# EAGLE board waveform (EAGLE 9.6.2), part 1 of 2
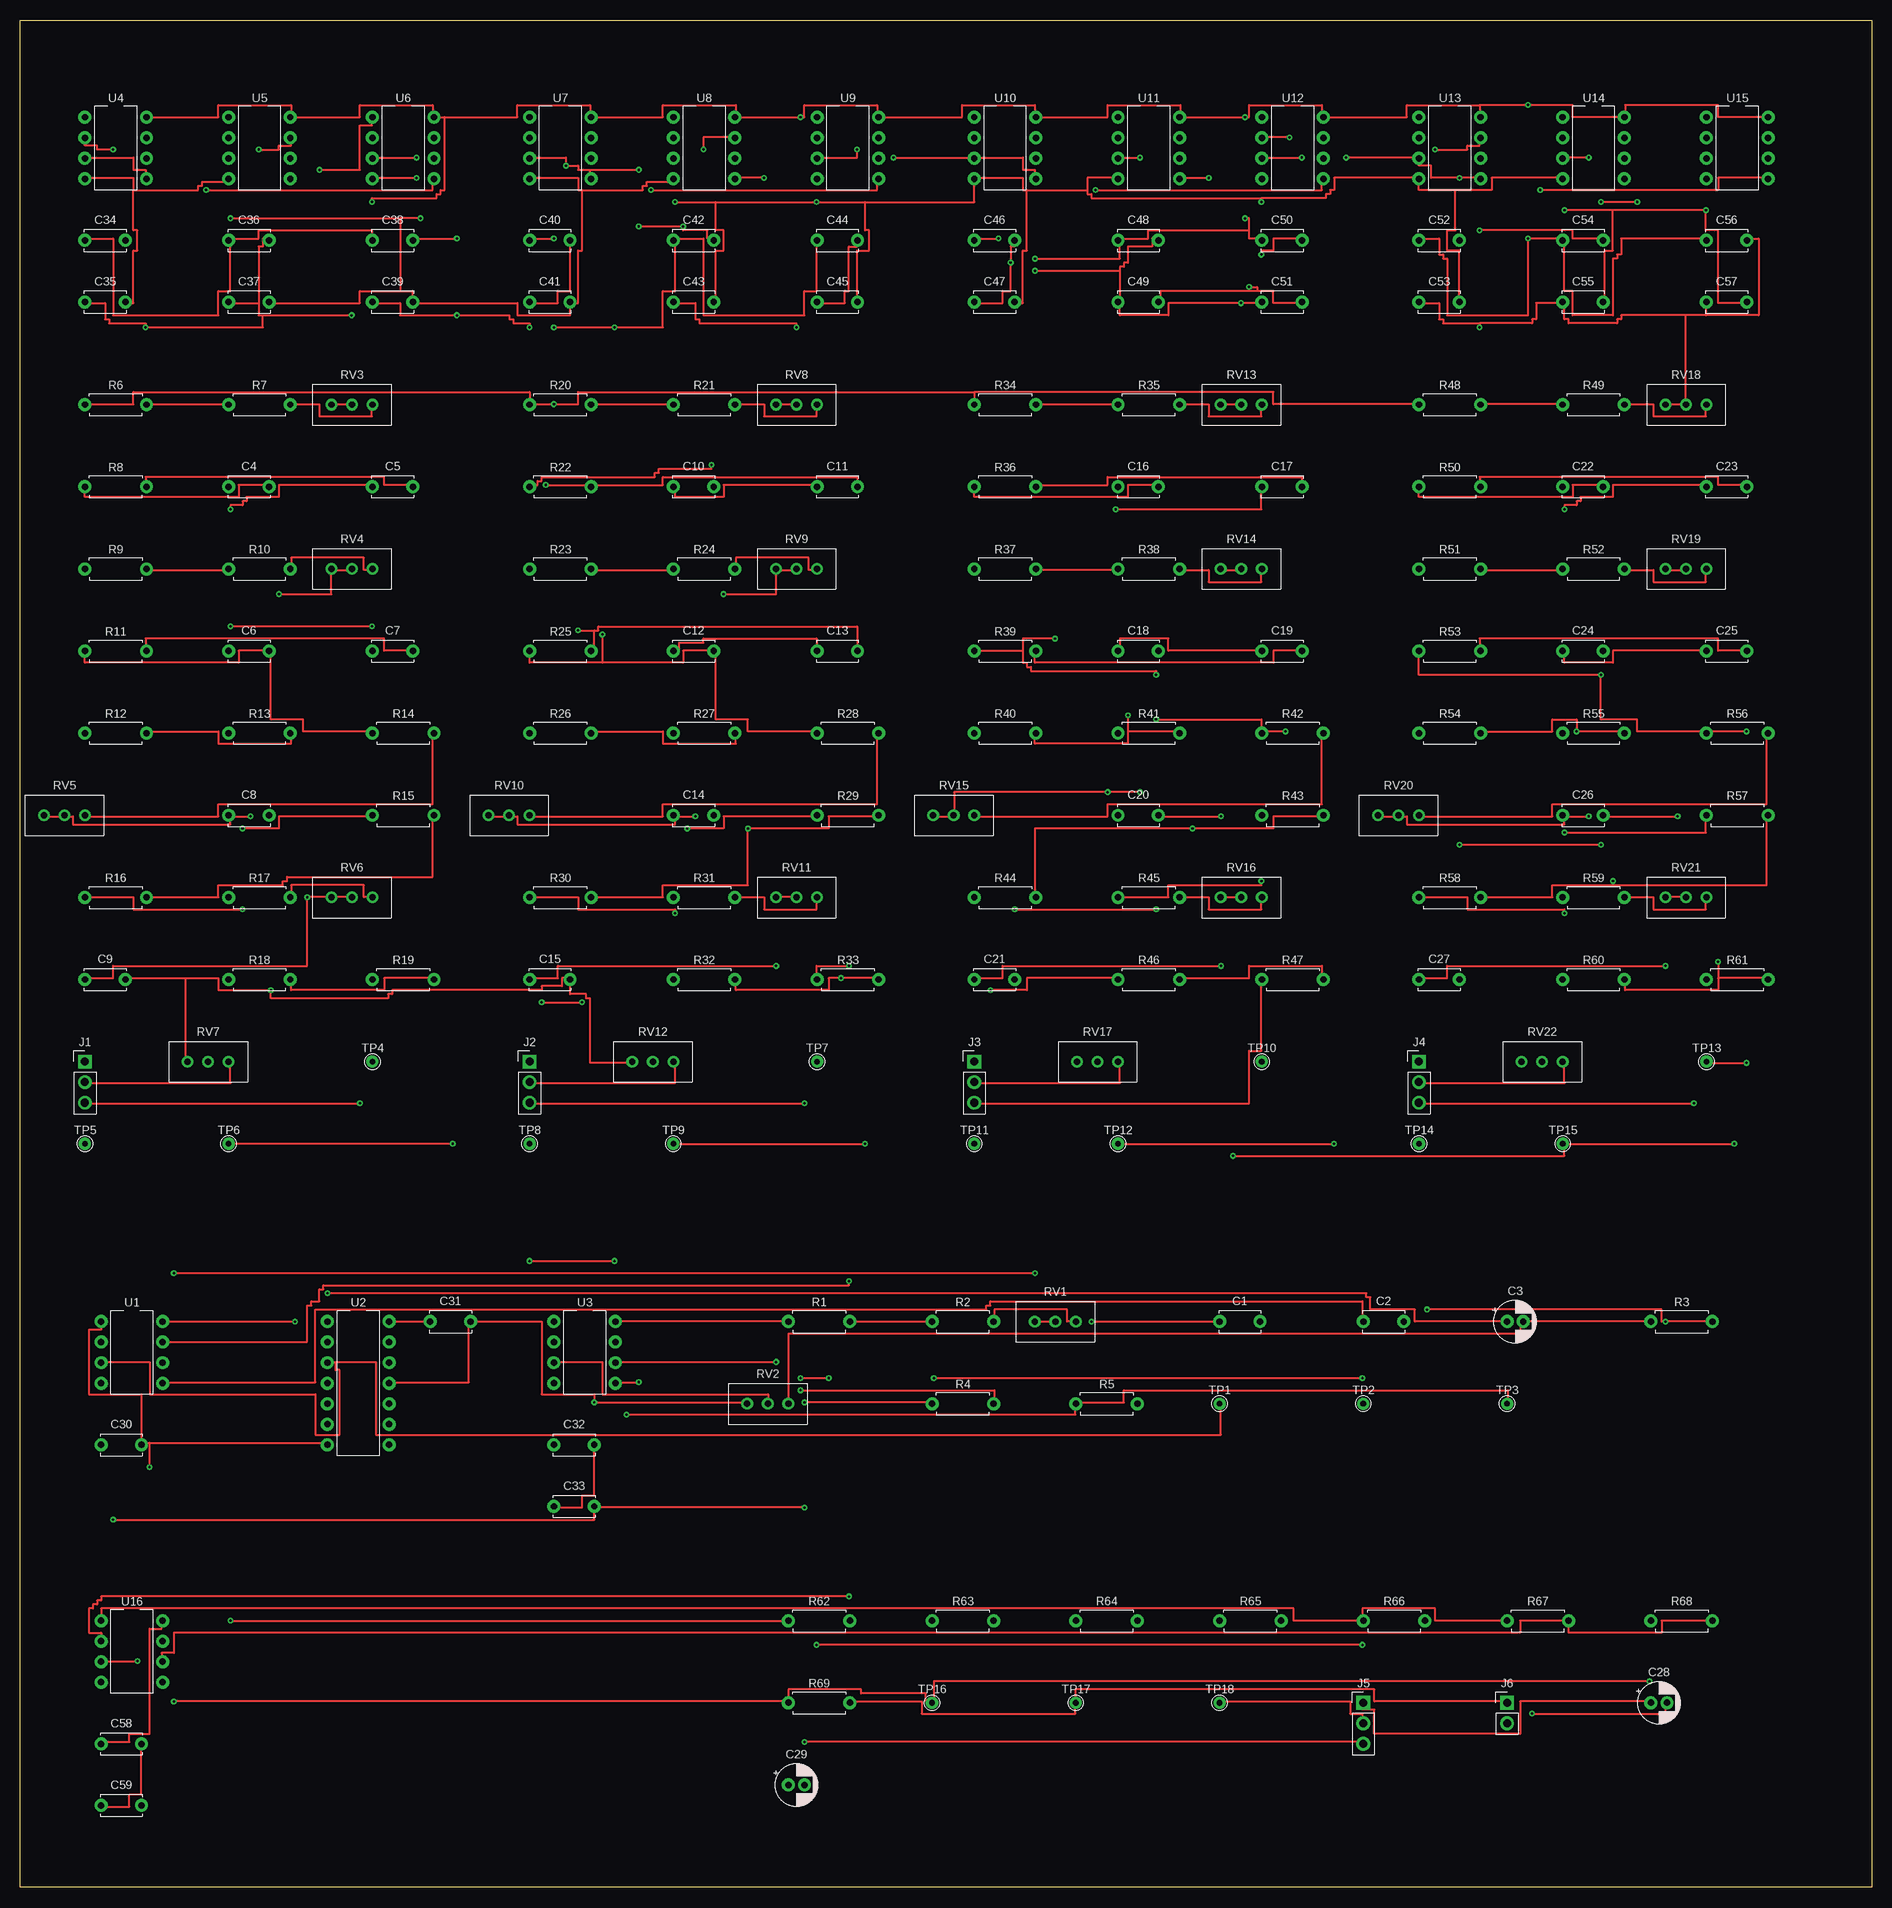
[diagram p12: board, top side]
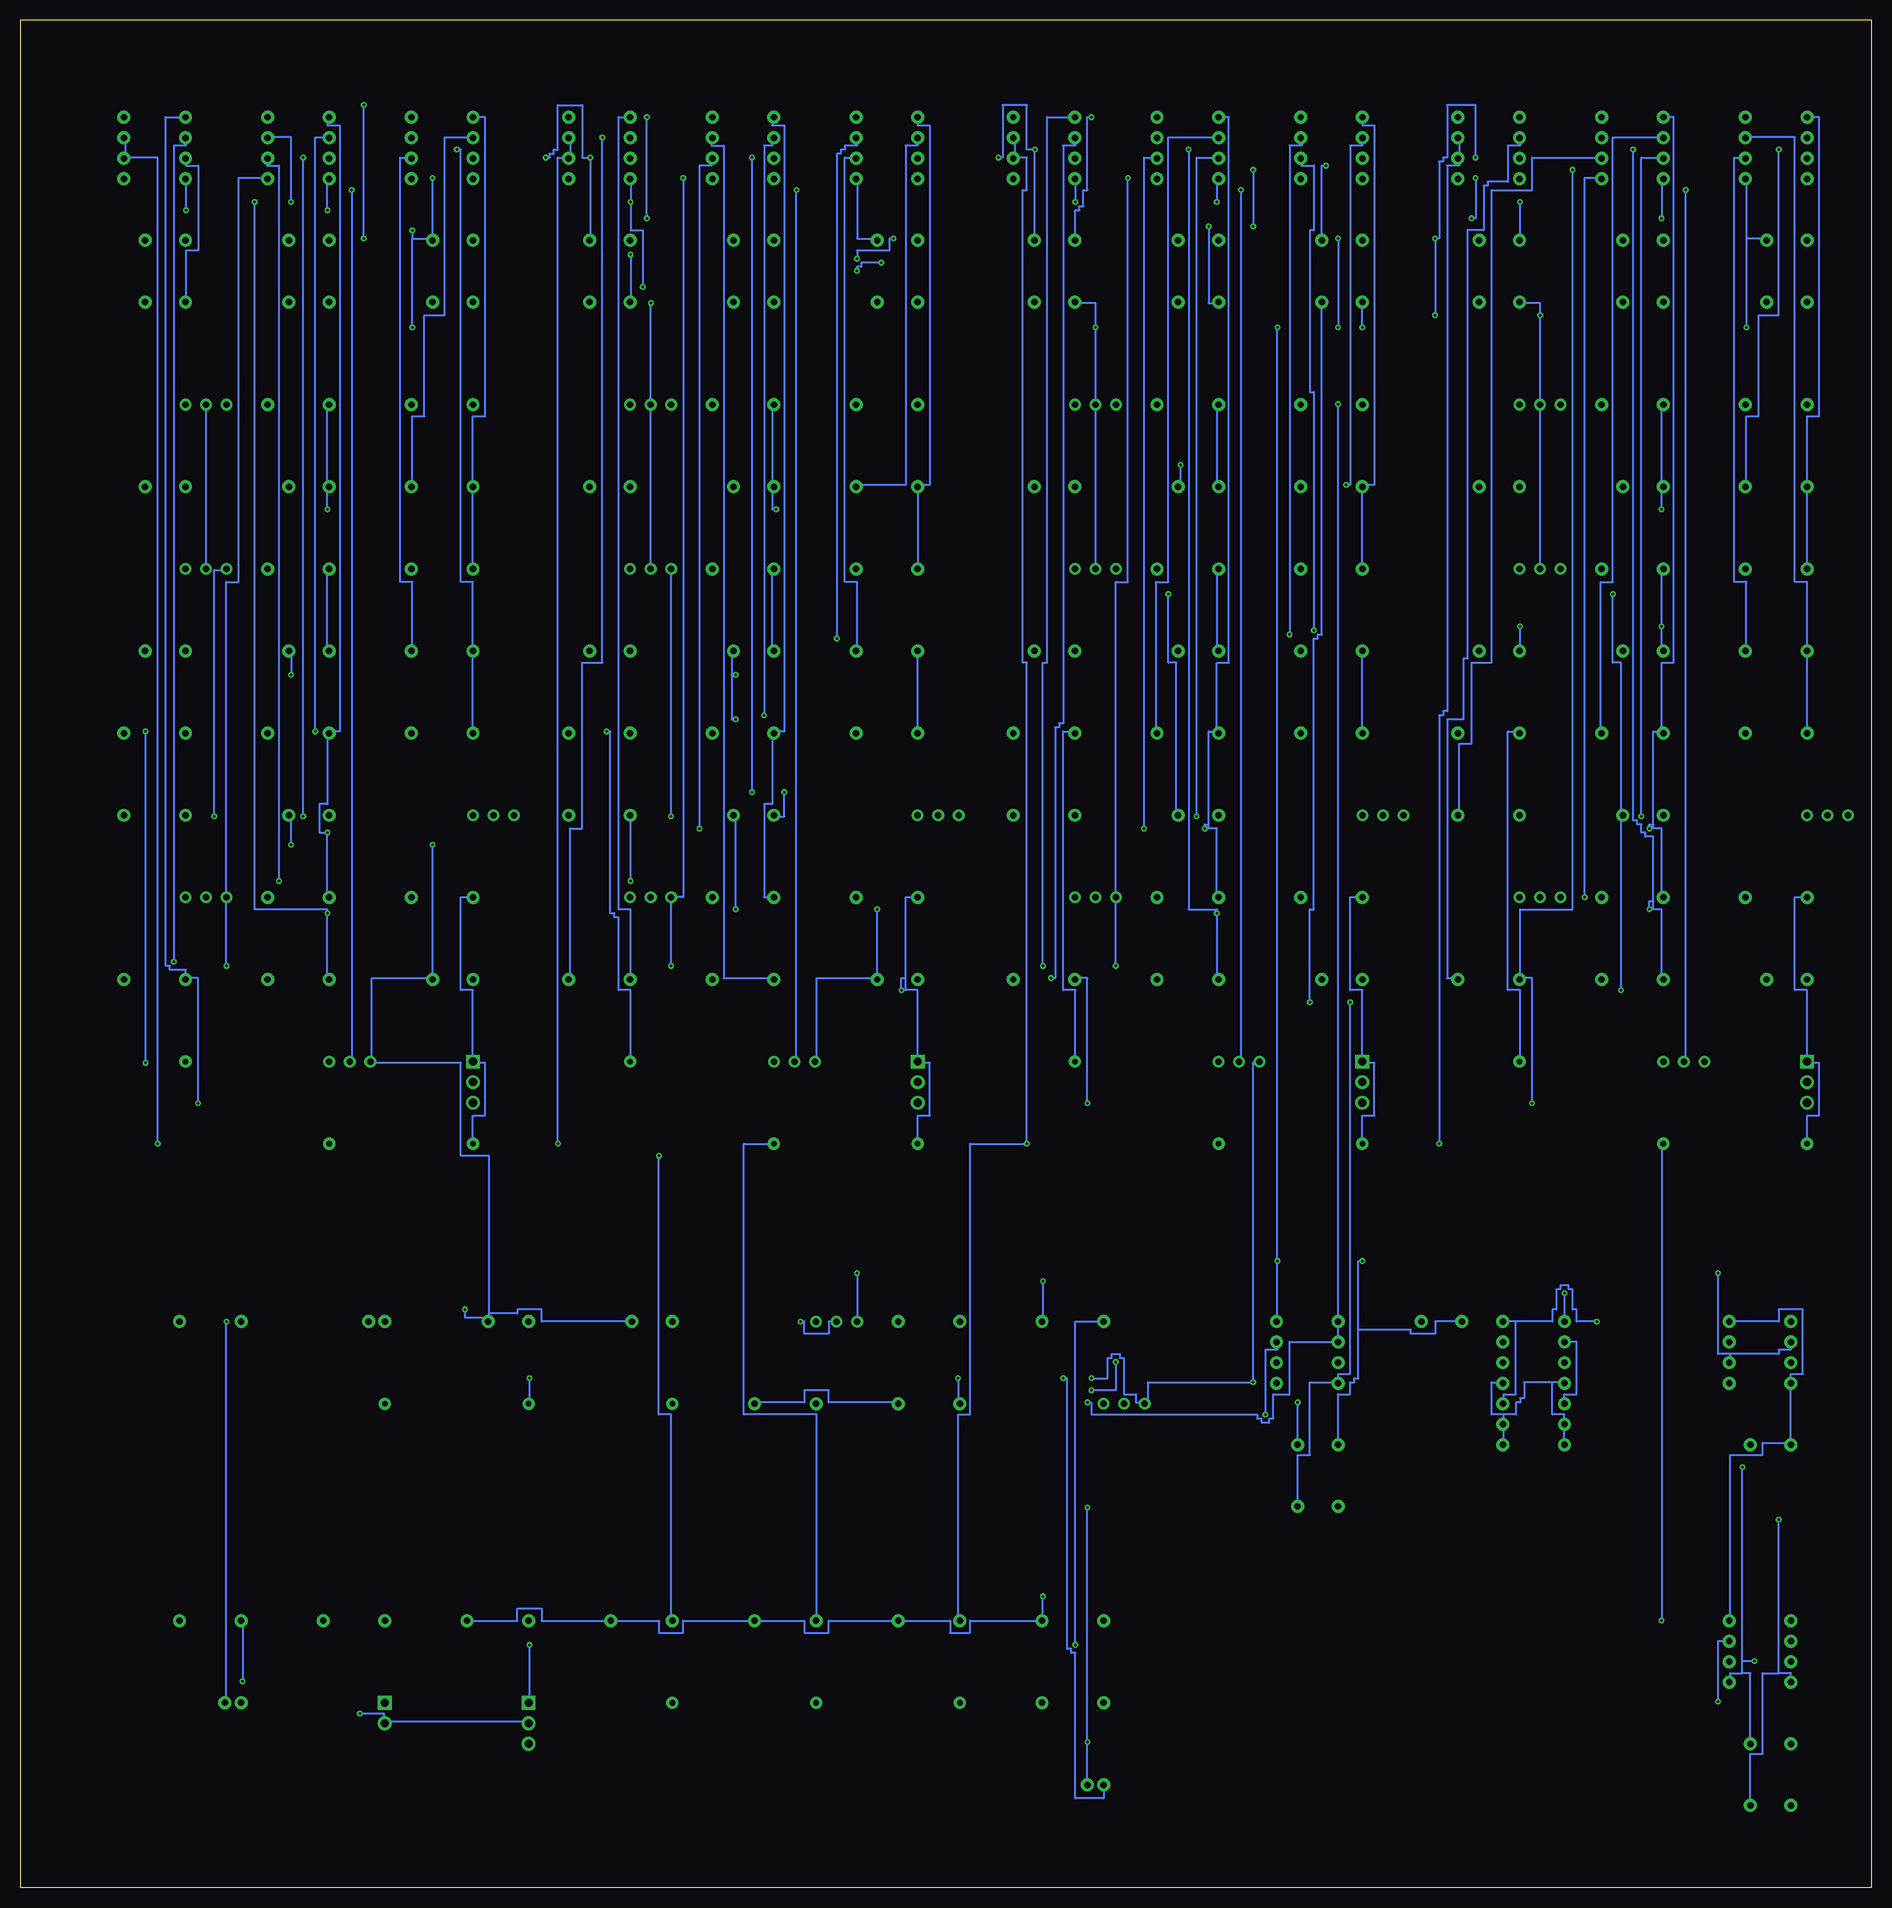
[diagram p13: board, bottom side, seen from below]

Size 229 x 231 mm. Coordinates in mm from the lower left corner, seen from the top.
Outline: 229,0 0,0 0,231 229,231 229,0
Copper layers (1*16): Top 0.035mm / Bottom 0.035mm
Design rules "Waveform_2layer_0.20mm": minimum track width 0.25mm, minimum drill 0.3mm, track to track 0.2mm, track to pad 0.2mm, pad to pad 0.2mm, via to via 0.2mm, copper to edge 0.5mm, stop-mask expansion 0.05mm
Net classes: 0 default: width 0.25 mm, drill 0.3 mm, clearance 0.2 mm

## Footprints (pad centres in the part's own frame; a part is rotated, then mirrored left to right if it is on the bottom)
C_Disc_D5.0mm_W2.5mm_P5.00mm = drill 0.8 pad 1.6 round: 1 0,0; 2 5,0
CP_Radial_D5.0mm_P2.00mm = drill 0.8 pad 1.6 round: 1 0,0; 2 2,0
PinHeader_1x03_P2.54mm_Vertical = drill 1 pad 1.7 square: 1 0,0 | drill 1 pad 1.7 round: 2 0,-2.54; 3 0,-5.08
PinHeader_1x02_P2.54mm_Vertical = drill 1 pad 1.7 square: 1 0,0 | drill 1 pad 1.7 round: 2 0,-2.54
R_Axial_DIN0207_L6.3mm_D2.5mm_P7.62mm_Horizontal = drill 0.8 pad 1.6 round: 1 0,0; 2 7.62,0
Potentiometer_Bourns_3296W_Vertical = drill 0.8 pad 1.44 round: 1 0,0; 2 -2.54,0; 3 -5.08,0
TestPoint_THTPad_D1.5mm_Drill0.7mm = drill 0.7 pad 1.5 round: 1 0,0
DIP-8_W7.62mm = drill 0.8 pad 1.6 round: 1 0,0; 2 0,-2.54; 3 0,-5.08; 4 0,-7.62; 5 7.62,-7.62; 6 7.62,-5.08; 7 7.62,-2.54; 8 7.62,0
DIP-14_W7.62mm = drill 0.8 pad 1.6 round: 1 0,0; 2 0,-2.54; 3 0,-5.08; 4 0,-7.62; 5 0,-10.16; 6 0,-12.7; 7 0,-15.24; 8 7.62,-15.24; 9 7.62,-12.7; 10 7.62,-10.16; 11 7.62,-7.62; 12 7.62,-5.08; 13 7.62,-2.54; 14 7.62,0

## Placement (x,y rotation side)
C1  10n  [C_Disc_D5.0mm_W2.5mm_P5.00mm]  148.34,70 0 top
C2  10n  [C_Disc_D5.0mm_W2.5mm_P5.00mm]  166.12,70 0 top
C3  10u/25V  [CP_Radial_D5.0mm_P2.00mm]  183.9,70 0 top
C4  10n  [C_Disc_D5.0mm_W2.5mm_P5.00mm]  25.78,173.28 0 top
C5  10n  [C_Disc_D5.0mm_W2.5mm_P5.00mm]  43.56,173.28 0 top
C6  10n  [C_Disc_D5.0mm_W2.5mm_P5.00mm]  25.78,152.96 0 top
C7  10n  [C_Disc_D5.0mm_W2.5mm_P5.00mm]  43.56,152.96 0 top
C8  10n  [C_Disc_D5.0mm_W2.5mm_P5.00mm]  25.78,132.64 0 top
C9  10n  [C_Disc_D5.0mm_W2.5mm_P5.00mm]  8,112.32 0 top
C10  3.3n  [C_Disc_D5.0mm_W2.5mm_P5.00mm]  80.78,173.28 0 top
C11  3.3n  [C_Disc_D5.0mm_W2.5mm_P5.00mm]  98.56,173.28 0 top
C12  3.3n  [C_Disc_D5.0mm_W2.5mm_P5.00mm]  80.78,152.96 0 top
C13  3.3n  [C_Disc_D5.0mm_W2.5mm_P5.00mm]  98.56,152.96 0 top
C14  3.3n  [C_Disc_D5.0mm_W2.5mm_P5.00mm]  80.78,132.64 0 top
C15  3.3n  [C_Disc_D5.0mm_W2.5mm_P5.00mm]  63,112.32 0 top
C16  2n  [C_Disc_D5.0mm_W2.5mm_P5.00mm]  135.78,173.28 0 top
C17  2n  [C_Disc_D5.0mm_W2.5mm_P5.00mm]  153.56,173.28 0 top
C18  2n  [C_Disc_D5.0mm_W2.5mm_P5.00mm]  135.78,152.96 0 top
C19  2n  [C_Disc_D5.0mm_W2.5mm_P5.00mm]  153.56,152.96 0 top
C20  2n  [C_Disc_D5.0mm_W2.5mm_P5.00mm]  135.78,132.64 0 top
C21  2n  [C_Disc_D5.0mm_W2.5mm_P5.00mm]  118,112.32 0 top
C22  1.5n  [C_Disc_D5.0mm_W2.5mm_P5.00mm]  190.78,173.28 0 top
C23  1.5n  [C_Disc_D5.0mm_W2.5mm_P5.00mm]  208.56,173.28 0 top
C24  1.5n  [C_Disc_D5.0mm_W2.5mm_P5.00mm]  190.78,152.96 0 top
C25  1.5n  [C_Disc_D5.0mm_W2.5mm_P5.00mm]  208.56,152.96 0 top
C26  1.5n  [C_Disc_D5.0mm_W2.5mm_P5.00mm]  190.78,132.64 0 top
C27  1.5n  [C_Disc_D5.0mm_W2.5mm_P5.00mm]  173,112.32 0 top
C28  47u/25V  [CP_Radial_D5.0mm_P2.00mm]  201.68,22.84 0 top
C29  47u/25V  [CP_Radial_D5.0mm_P2.00mm]  95,12.68 0 top
C30  100n  [C_Disc_D5.0mm_W2.5mm_P5.00mm]  10,54.76 0 top
C31  100n  [C_Disc_D5.0mm_W2.5mm_P5.00mm]  50.7,70 0 top
C32  100n  [C_Disc_D5.0mm_W2.5mm_P5.00mm]  66,54.76 0 top
C33  100n  [C_Disc_D5.0mm_W2.5mm_P5.00mm]  66,47.14 0 top
C34  100n  [C_Disc_D5.0mm_W2.5mm_P5.00mm]  8,203.76 0 top
C35  100n  [C_Disc_D5.0mm_W2.5mm_P5.00mm]  8,196.14 0 top
C36  100n  [C_Disc_D5.0mm_W2.5mm_P5.00mm]  25.78,203.76 0 top
C37  100n  [C_Disc_D5.0mm_W2.5mm_P5.00mm]  25.78,196.14 0 top
C38  100n  [C_Disc_D5.0mm_W2.5mm_P5.00mm]  43.56,203.76 0 top
C39  100n  [C_Disc_D5.0mm_W2.5mm_P5.00mm]  43.56,196.14 0 top
C40  100n  [C_Disc_D5.0mm_W2.5mm_P5.00mm]  63,203.76 0 top
C41  100n  [C_Disc_D5.0mm_W2.5mm_P5.00mm]  63,196.14 0 top
C42  100n  [C_Disc_D5.0mm_W2.5mm_P5.00mm]  80.78,203.76 0 top
C43  100n  [C_Disc_D5.0mm_W2.5mm_P5.00mm]  80.78,196.14 0 top
C44  100n  [C_Disc_D5.0mm_W2.5mm_P5.00mm]  98.56,203.76 0 top
C45  100n  [C_Disc_D5.0mm_W2.5mm_P5.00mm]  98.56,196.14 0 top
C46  100n  [C_Disc_D5.0mm_W2.5mm_P5.00mm]  118,203.76 0 top
C47  100n  [C_Disc_D5.0mm_W2.5mm_P5.00mm]  118,196.14 0 top
C48  100n  [C_Disc_D5.0mm_W2.5mm_P5.00mm]  135.78,203.76 0 top
C49  100n  [C_Disc_D5.0mm_W2.5mm_P5.00mm]  135.78,196.14 0 top
C50  100n  [C_Disc_D5.0mm_W2.5mm_P5.00mm]  153.56,203.76 0 top
C51  100n  [C_Disc_D5.0mm_W2.5mm_P5.00mm]  153.56,196.14 0 top
C52  100n  [C_Disc_D5.0mm_W2.5mm_P5.00mm]  173,203.76 0 top
C53  100n  [C_Disc_D5.0mm_W2.5mm_P5.00mm]  173,196.14 0 top
C54  100n  [C_Disc_D5.0mm_W2.5mm_P5.00mm]  190.78,203.76 0 top
C55  100n  [C_Disc_D5.0mm_W2.5mm_P5.00mm]  190.78,196.14 0 top
C56  100n  [C_Disc_D5.0mm_W2.5mm_P5.00mm]  208.56,203.76 0 top
C57  100n  [C_Disc_D5.0mm_W2.5mm_P5.00mm]  208.56,196.14 0 top
C58  100n  [C_Disc_D5.0mm_W2.5mm_P5.00mm]  10,17.76 0 top
C59  100n  [C_Disc_D5.0mm_W2.5mm_P5.00mm]  10,10.14 0 top
J1  PHASE_POLARITY  [PinHeader_1x03_P2.54mm_Vertical]  8,102.16 0 top
J2  PHASE_POLARITY  [PinHeader_1x03_P2.54mm_Vertical]  63,102.16 0 top
J3  PHASE_POLARITY  [PinHeader_1x03_P2.54mm_Vertical]  118,102.16 0 top
J4  PHASE_POLARITY  [PinHeader_1x03_P2.54mm_Vertical]  173,102.16 0 top
J5  POWER_12V  [PinHeader_1x03_P2.54mm_Vertical]  166.12,22.84 0 top
J6  WAVE_OUT  [PinHeader_1x02_P2.54mm_Vertical]  183.9,22.84 0 top
R1  10k  [R_Axial_DIN0207_L6.3mm_D2.5mm_P7.62mm_Horizontal]  95,70 0 top
R2  27k  [R_Axial_DIN0207_L6.3mm_D2.5mm_P7.62mm_Horizontal]  112.78,70 0 top
R3  1M  [R_Axial_DIN0207_L6.3mm_D2.5mm_P7.62mm_Horizontal]  201.68,70 0 top
R4  100k  [R_Axial_DIN0207_L6.3mm_D2.5mm_P7.62mm_Horizontal]  112.78,59.84 0 top
R5  100k  [R_Axial_DIN0207_L6.3mm_D2.5mm_P7.62mm_Horizontal]  130.56,59.84 0 top
R6  220k  [R_Axial_DIN0207_L6.3mm_D2.5mm_P7.62mm_Horizontal]  8,183.44 0 top
R7  430  [R_Axial_DIN0207_L6.3mm_D2.5mm_P7.62mm_Horizontal]  25.78,183.44 0 top
R8  470k  [R_Axial_DIN0207_L6.3mm_D2.5mm_P7.62mm_Horizontal]  8,173.28 0 top
R9  220k  [R_Axial_DIN0207_L6.3mm_D2.5mm_P7.62mm_Horizontal]  8,163.12 0 top
R10  430  [R_Axial_DIN0207_L6.3mm_D2.5mm_P7.62mm_Horizontal]  25.78,163.12 0 top
R11  470k  [R_Axial_DIN0207_L6.3mm_D2.5mm_P7.62mm_Horizontal]  8,152.96 0 top
R12  10k  [R_Axial_DIN0207_L6.3mm_D2.5mm_P7.62mm_Horizontal]  8,142.8 0 top
R13  10k  [R_Axial_DIN0207_L6.3mm_D2.5mm_P7.62mm_Horizontal]  25.78,142.8 0 top
R14  100  [R_Axial_DIN0207_L6.3mm_D2.5mm_P7.62mm_Horizontal]  43.56,142.8 0 top
R15  10k  [R_Axial_DIN0207_L6.3mm_D2.5mm_P7.62mm_Horizontal]  43.56,132.64 0 top
R16  10k  [R_Axial_DIN0207_L6.3mm_D2.5mm_P7.62mm_Horizontal]  8,122.48 0 top
R17  100  [R_Axial_DIN0207_L6.3mm_D2.5mm_P7.62mm_Horizontal]  25.78,122.48 0 top
R18  10k  [R_Axial_DIN0207_L6.3mm_D2.5mm_P7.62mm_Horizontal]  25.78,112.32 0 top
R19  10k  [R_Axial_DIN0207_L6.3mm_D2.5mm_P7.62mm_Horizontal]  43.56,112.32 0 top
R20  220k  [R_Axial_DIN0207_L6.3mm_D2.5mm_P7.62mm_Horizontal]  63,183.44 0 top
R21  430  [R_Axial_DIN0207_L6.3mm_D2.5mm_P7.62mm_Horizontal]  80.78,183.44 0 top
R22  470k  [R_Axial_DIN0207_L6.3mm_D2.5mm_P7.62mm_Horizontal]  63,173.28 0 top
R23  220k  [R_Axial_DIN0207_L6.3mm_D2.5mm_P7.62mm_Horizontal]  63,163.12 0 top
R24  430  [R_Axial_DIN0207_L6.3mm_D2.5mm_P7.62mm_Horizontal]  80.78,163.12 0 top
R25  470k  [R_Axial_DIN0207_L6.3mm_D2.5mm_P7.62mm_Horizontal]  63,152.96 0 top
R26  10k  [R_Axial_DIN0207_L6.3mm_D2.5mm_P7.62mm_Horizontal]  63,142.8 0 top
R27  10k  [R_Axial_DIN0207_L6.3mm_D2.5mm_P7.62mm_Horizontal]  80.78,142.8 0 top
R28  100  [R_Axial_DIN0207_L6.3mm_D2.5mm_P7.62mm_Horizontal]  98.56,142.8 0 top
R29  10k  [R_Axial_DIN0207_L6.3mm_D2.5mm_P7.62mm_Horizontal]  98.56,132.64 0 top
R30  10k  [R_Axial_DIN0207_L6.3mm_D2.5mm_P7.62mm_Horizontal]  63,122.48 0 top
R31  100  [R_Axial_DIN0207_L6.3mm_D2.5mm_P7.62mm_Horizontal]  80.78,122.48 0 top
R32  10k  [R_Axial_DIN0207_L6.3mm_D2.5mm_P7.62mm_Horizontal]  80.78,112.32 0 top
R33  10k  [R_Axial_DIN0207_L6.3mm_D2.5mm_P7.62mm_Horizontal]  98.56,112.32 0 top
R34  220k  [R_Axial_DIN0207_L6.3mm_D2.5mm_P7.62mm_Horizontal]  118,183.44 0 top
R35  430  [R_Axial_DIN0207_L6.3mm_D2.5mm_P7.62mm_Horizontal]  135.78,183.44 0 top
R36  470k  [R_Axial_DIN0207_L6.3mm_D2.5mm_P7.62mm_Horizontal]  118,173.28 0 top
R37  220k  [R_Axial_DIN0207_L6.3mm_D2.5mm_P7.62mm_Horizontal]  118,163.12 0 top
R38  430  [R_Axial_DIN0207_L6.3mm_D2.5mm_P7.62mm_Horizontal]  135.78,163.12 0 top
R39  470k  [R_Axial_DIN0207_L6.3mm_D2.5mm_P7.62mm_Horizontal]  118,152.96 0 top
R40  10k  [R_Axial_DIN0207_L6.3mm_D2.5mm_P7.62mm_Horizontal]  118,142.8 0 top
R41  10k  [R_Axial_DIN0207_L6.3mm_D2.5mm_P7.62mm_Horizontal]  135.78,142.8 0 top
R42  100  [R_Axial_DIN0207_L6.3mm_D2.5mm_P7.62mm_Horizontal]  153.56,142.8 0 top
R43  10k  [R_Axial_DIN0207_L6.3mm_D2.5mm_P7.62mm_Horizontal]  153.56,132.64 0 top
R44  10k  [R_Axial_DIN0207_L6.3mm_D2.5mm_P7.62mm_Horizontal]  118,122.48 0 top
R45  100  [R_Axial_DIN0207_L6.3mm_D2.5mm_P7.62mm_Horizontal]  135.78,122.48 0 top
R46  10k  [R_Axial_DIN0207_L6.3mm_D2.5mm_P7.62mm_Horizontal]  135.78,112.32 0 top
R47  10k  [R_Axial_DIN0207_L6.3mm_D2.5mm_P7.62mm_Horizontal]  153.56,112.32 0 top
R48  220k  [R_Axial_DIN0207_L6.3mm_D2.5mm_P7.62mm_Horizontal]  173,183.44 0 top
R49  430  [R_Axial_DIN0207_L6.3mm_D2.5mm_P7.62mm_Horizontal]  190.78,183.44 0 top
R50  470k  [R_Axial_DIN0207_L6.3mm_D2.5mm_P7.62mm_Horizontal]  173,173.28 0 top
R51  220k  [R_Axial_DIN0207_L6.3mm_D2.5mm_P7.62mm_Horizontal]  173,163.12 0 top
R52  430  [R_Axial_DIN0207_L6.3mm_D2.5mm_P7.62mm_Horizontal]  190.78,163.12 0 top
R53  470k  [R_Axial_DIN0207_L6.3mm_D2.5mm_P7.62mm_Horizontal]  173,152.96 0 top
R54  10k  [R_Axial_DIN0207_L6.3mm_D2.5mm_P7.62mm_Horizontal]  173,142.8 0 top
R55  10k  [R_Axial_DIN0207_L6.3mm_D2.5mm_P7.62mm_Horizontal]  190.78,142.8 0 top
R56  100  [R_Axial_DIN0207_L6.3mm_D2.5mm_P7.62mm_Horizontal]  208.56,142.8 0 top
R57  10k  [R_Axial_DIN0207_L6.3mm_D2.5mm_P7.62mm_Horizontal]  208.56,132.64 0 top
R58  10k  [R_Axial_DIN0207_L6.3mm_D2.5mm_P7.62mm_Horizontal]  173,122.48 0 top
R59  100  [R_Axial_DIN0207_L6.3mm_D2.5mm_P7.62mm_Horizontal]  190.78,122.48 0 top
R60  10k  [R_Axial_DIN0207_L6.3mm_D2.5mm_P7.62mm_Horizontal]  190.78,112.32 0 top
R61  10k  [R_Axial_DIN0207_L6.3mm_D2.5mm_P7.62mm_Horizontal]  208.56,112.32 0 top
R62  100k  [R_Axial_DIN0207_L6.3mm_D2.5mm_P7.62mm_Horizontal]  95,33 0 top
R63  100k  [R_Axial_DIN0207_L6.3mm_D2.5mm_P7.62mm_Horizontal]  112.78,33 0 top
R64  100k  [R_Axial_DIN0207_L6.3mm_D2.5mm_P7.62mm_Horizontal]  130.56,33 0 top
R65  100k  [R_Axial_DIN0207_L6.3mm_D2.5mm_P7.62mm_Horizontal]  148.34,33 0 top
R66  100k  [R_Axial_DIN0207_L6.3mm_D2.5mm_P7.62mm_Horizontal]  166.12,33 0 top
R67  100k  [R_Axial_DIN0207_L6.3mm_D2.5mm_P7.62mm_Horizontal]  183.9,33 0 top
R68  100k  [R_Axial_DIN0207_L6.3mm_D2.5mm_P7.62mm_Horizontal]  201.68,33 0 top
R69  100  [R_Axial_DIN0207_L6.3mm_D2.5mm_P7.62mm_Horizontal]  95,22.84 0 top
RV1  20k  [Potentiometer_Bourns_3296W_Vertical]  130.56,70 0 top
RV2  100k  [Potentiometer_Bourns_3296W_Vertical]  95,59.84 0 top
RV3  200  [Potentiometer_Bourns_3296W_Vertical]  43.56,183.44 0 top
RV4  200  [Potentiometer_Bourns_3296W_Vertical]  43.56,163.12 0 top
RV5  200k  [Potentiometer_Bourns_3296W_Vertical]  8,132.64 0 top
RV6  200k  [Potentiometer_Bourns_3296W_Vertical]  43.56,122.48 0 top
RV7  10k  [Potentiometer_Bourns_3296W_Vertical]  25.78,102.16 0 top
RV8  200  [Potentiometer_Bourns_3296W_Vertical]  98.56,183.44 0 top
RV9  200  [Potentiometer_Bourns_3296W_Vertical]  98.56,163.12 0 top
RV10  200k  [Potentiometer_Bourns_3296W_Vertical]  63,132.64 0 top
RV11  200k  [Potentiometer_Bourns_3296W_Vertical]  98.56,122.48 0 top
RV12  10k  [Potentiometer_Bourns_3296W_Vertical]  80.78,102.16 0 top
RV13  200  [Potentiometer_Bourns_3296W_Vertical]  153.56,183.44 0 top
RV14  200  [Potentiometer_Bourns_3296W_Vertical]  153.56,163.12 0 top
RV15  200k  [Potentiometer_Bourns_3296W_Vertical]  118,132.64 0 top
RV16  200k  [Potentiometer_Bourns_3296W_Vertical]  153.56,122.48 0 top
RV17  10k  [Potentiometer_Bourns_3296W_Vertical]  135.78,102.16 0 top
RV18  200  [Potentiometer_Bourns_3296W_Vertical]  208.56,183.44 0 top
RV19  200  [Potentiometer_Bourns_3296W_Vertical]  208.56,163.12 0 top
RV20  200k  [Potentiometer_Bourns_3296W_Vertical]  173,132.64 0 top
RV21  200k  [Potentiometer_Bourns_3296W_Vertical]  208.56,122.48 0 top
RV22  10k  [Potentiometer_Bourns_3296W_Vertical]  190.78,102.16 0 top
TP1  CLOCK_2K  [TestPoint_THTPad_D1.5mm_Drill0.7mm]  148.34,59.84 0 top
TP2  SQ  [TestPoint_THTPad_D1.5mm_Drill0.7mm]  166.12,59.84 0 top
TP3  SQ_INV  [TestPoint_THTPad_D1.5mm_Drill0.7mm]  183.9,59.84 0 top
TP4  H1_BPF2  [TestPoint_THTPad_D1.5mm_Drill0.7mm]  43.56,102.16 0 top
TP5  H1_AP2  [TestPoint_THTPad_D1.5mm_Drill0.7mm]  8,92 0 top
TP6  H1_OUT  [TestPoint_THTPad_D1.5mm_Drill0.7mm]  25.78,92 0 top
TP7  H3_BPF2  [TestPoint_THTPad_D1.5mm_Drill0.7mm]  98.56,102.16 0 top
TP8  H3_AP2  [TestPoint_THTPad_D1.5mm_Drill0.7mm]  63,92 0 top
TP9  H3_OUT  [TestPoint_THTPad_D1.5mm_Drill0.7mm]  80.78,92 0 top
TP10  H5_BPF2  [TestPoint_THTPad_D1.5mm_Drill0.7mm]  153.56,102.16 0 top
TP11  H5_AP2  [TestPoint_THTPad_D1.5mm_Drill0.7mm]  118,92 0 top
TP12  H5_OUT  [TestPoint_THTPad_D1.5mm_Drill0.7mm]  135.78,92 0 top
TP13  H7_BPF2  [TestPoint_THTPad_D1.5mm_Drill0.7mm]  208.56,102.16 0 top
TP14  H7_AP2  [TestPoint_THTPad_D1.5mm_Drill0.7mm]  173,92 0 top
TP15  H7_OUT  [TestPoint_THTPad_D1.5mm_Drill0.7mm]  190.78,92 0 top
TP16  SUM_RAW  [TestPoint_THTPad_D1.5mm_Drill0.7mm]  112.78,22.84 0 top
TP17  OUT  [TestPoint_THTPad_D1.5mm_Drill0.7mm]  130.56,22.84 0 top
TP18  GND  [TestPoint_THTPad_D1.5mm_Drill0.7mm]  148.34,22.84 0 top
U1  NE555P  [DIP-8_W7.62mm]  10,70 0 top
U2  CD4013BE  [DIP-14_W7.62mm]  38,70 0 top
U3  TL082CP  [DIP-8_W7.62mm]  66,70 0 top
U4  TL082CP  [DIP-8_W7.62mm]  8,219 0 top
U5  TL082CP  [DIP-8_W7.62mm]  25.78,219 0 top
U6  TL082CP  [DIP-8_W7.62mm]  43.56,219 0 top
U7  TL082CP  [DIP-8_W7.62mm]  63,219 0 top
U8  TL082CP  [DIP-8_W7.62mm]  80.78,219 0 top
U9  TL082CP  [DIP-8_W7.62mm]  98.56,219 0 top
U10  TL082CP  [DIP-8_W7.62mm]  118,219 0 top
U11  TL082CP  [DIP-8_W7.62mm]  135.78,219 0 top
U12  TL082CP  [DIP-8_W7.62mm]  153.56,219 0 top
U13  TL082CP  [DIP-8_W7.62mm]  173,219 0 top
U14  TL082CP  [DIP-8_W7.62mm]  190.78,219 0 top
U15  TL082CP  [DIP-8_W7.62mm]  208.56,219 0 top
U16  TL082CP  [DIP-8_W7.62mm]  10,33 0 top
